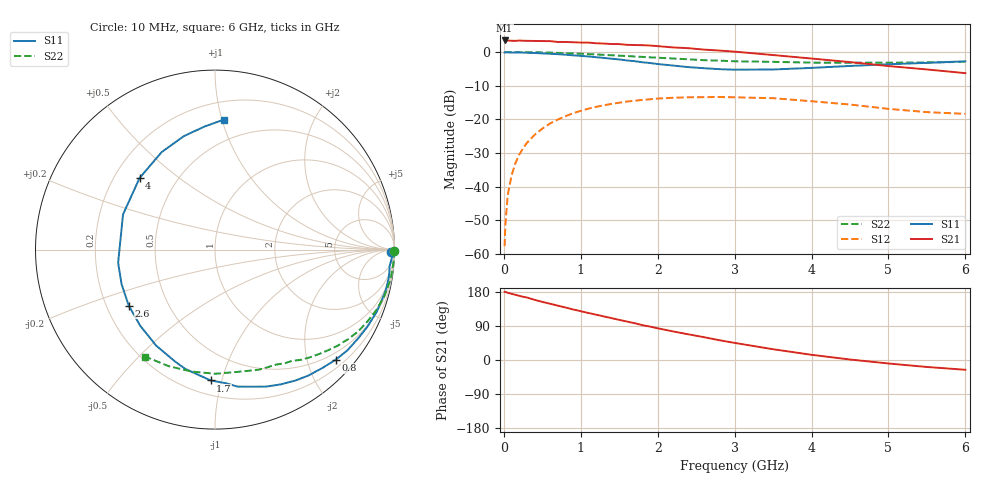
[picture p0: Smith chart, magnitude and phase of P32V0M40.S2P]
! SIEMENS Small Signal Semiconductors
! BFP181
! Si NPN RF Bipolar Junction Transistor in SOT143
! VCE = 2 V  IC = 0.4 mA
! Common Emitter S-Parameters:  March  1996
# GHz  S  MA  R  50
!  f  S11  S21  S12  S22
! GHz  MAG  ANG  MAG  ANG  MAG  ANG  MAG  ANG
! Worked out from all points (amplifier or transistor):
!   36 points, 10 MHz to 6 GHz, reference 50 ohm
!   highest |S21| = 3.4 dB at 10 MHz (marker M1)
!   |S21| within 3 dB of that: start of sweep to 2.803 GHz
!   unconditionally stable (mu >= 1): 3.81 GHz to end of sweep
!   at 250 MHz: K = 0.08, MSG = 16.0 dB, |S12| = -28.6 dB
!   at 1.4 GHz: K = 0.43, MSG = 8.9 dB, |S12| = -15.5 dB
!   at 6 GHz: K = 1.53, MAG = 1.8 dB, |S12| = -18.4 dB
!   S11 on the Smith chart (normalised r, x): 10 MHz: 77, -53; 800 MHz: 0.35, -2.54; 1.7 GHz: 0.30, -0.92; 2.6 GHz: 0.29, -0.27; 4 GHz: 0.31, +0.37; 6 GHz: 0.33, +1.01
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0.01  0.9825 -0.7  1.481 179.8  0.0013 83.7  0.9989 -0.3
0.02  0.9831 -1.1  1.469 179.8  0.0027 84.8  0.9984 -0.5
0.05  0.9867 -2.6  1.477 177.4  0.0074 90.0  0.9983 -1.3
0.1  0.9771 -5.4  1.465 174.7  0.0146 83.7  0.9988 -2.6
0.15  0.9801 -8.1  1.46 172.1  0.0222 84.1  0.9971 -3.9
0.2  0.9797 -10.5  1.477 169.4  0.0297 82.9  0.9958 -5.2
0.3  0.9723 -15.9  1.462 164.9  0.0445 78.3  0.9935 -7.9
0.4  0.9653 -21.0  1.456 158.8  0.0586 74.4  0.9895 -10.4
0.6  0.9387 -31.8  1.448 148.6  0.0863 66.7  0.9775 -15.6
0.8  0.9102 -42.4  1.406 138.6  0.1107 59.3  0.9599 -20.5
1.1  0.8563 -58.4  1.377 124.0  0.1437 48.6  0.9282 -27.5
1.5  0.774 -80.6  1.308 105.9  0.176 35.4  0.8794 -36.0
1.7  0.7295 -91.9  1.266 97.1  0.1882 29.6  0.8548 -39.9
1.9  0.6846 -104.1  1.245 88.2  0.198 23.7  0.8307 -43.6
2.2  0.6274 -121.5  1.167 75.4  0.2086 15.8  0.7988 -48.8
2.6  0.573 -147.0  1.083 60.3  0.2127 6.3  0.754 -55.3
3  0.5446 -172.3  1.01 45.1  0.2117 -3.1  0.7265 -61.8
3.5  0.5485 159.1  0.899 28.4  0.2055 -12.5  0.7125 -69.9
4  0.5794 136.5  0.798 13.7  0.1851 -20.0  0.6931 -79.4
4.5  0.6192 118.7  0.706 1.3  0.1653 -25.8  0.6918 -89.9
5.5  0.6883 94.8  0.549 -18.4  0.1275 -24.0  0.699 -111.7
6  0.7259 86.1  0.484 -25.8  0.1202 -19.2  0.7113 -123.0
